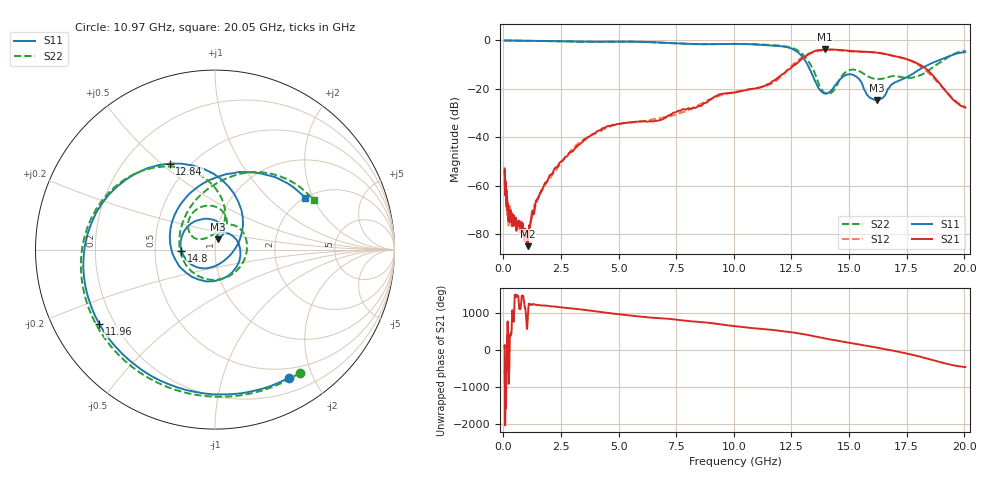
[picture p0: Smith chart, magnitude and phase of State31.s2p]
# Hz S DB R 50
!freq MagS11 AngS11 MagS21 AngS21 MagS12 AngS12 MagS22 AngS22
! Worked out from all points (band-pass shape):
!   1601 points, 50 MHz to 20.05 GHz, reference 50 ohm
!   highest |S21| = -3.69 dB at 13.94 GHz (marker M1); lowest = -85.1 dB at 1.047 GHz (marker M2)
!   |S21| within 3 dB of the highest: 13.1 GHz to 17.09 GHz (3.995 GHz wide, 26.5 % of centre)
!   lowest |S11| = -24.6 dB at 16.19 GHz (marker M3), VSWR 1.12, Z = 51.1 + j5.85 ohm
!   |S11| at or under -10 dB: 13.2 GHz to 18.45 GHz (5.254 GHz wide, 33.2 % of centre)
!   |S22| runs from -22.1 to 0.0 dB; largest |S21 - S12| = 0.044
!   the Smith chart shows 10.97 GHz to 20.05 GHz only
!   S11 on the Smith chart (normalised r, x): 10.97 GHz: 0.37, -1.66; 11.96 GHz: 0.14, -0.29; 12.84 GHz: 0.39, +0.53; 14.8 GHz: 0.69, -0.01; 20.05 GHz: 2.00, +1.74
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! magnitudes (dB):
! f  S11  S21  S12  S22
! 50 MHz  0.0  -55.4  -52.4  0.0
! 58.96 MHz  0.0  -55.1  -58.3  0.0
! 78.67 MHz  0.0  -62.8  -59.4  0.0
! 87.38 MHz  0.0  -59.9  -58.9  0.0
! 135.9 MHz  0.0  -66.6  -66.5  0.0
! 222.1 MHz  0.0  -74.2  -76.0  0.0
! 253.2 MHz  0.0  -71.2  -69.1  0.0
! 369.6 MHz  0.0  -76.4  -73.3  0.0
! 457.6 MHz  0.0  -73.5  -75.3  0.0
! 1.005 GHz  -0.1  -82.7  -80.7  -0.1
! 1.047 GHz  -0.1  -85.1  -81.0  -0.1
! 2.722 GHz  -0.3  -48.1  -48.0  -0.4
! 4.397 GHz  -0.5  -36.1  -36.5  -0.6
! 7.402 GHz  -1.1  -29.8  -30.8  -1.1
! 10.97 GHz  -1.7  -19.8  -19.7  -1.6
! 11.96 GHz  -2.3  -15.1  -15.7  -2.1
! 12.84 GHz  -5.3  -8.6  -7.8  -4.5
! 13.94 GHz  -22.0  -3.7  -3.9  -21.6
! 14.8 GHz  -14.6  -4.1  -4.3  -13.5
! 16.19 GHz  -24.6  -5.0  -5.0  -16.0
! 18.05 GHz  -12.0  -9.9  -10.4  -14.5
! 20.05 GHz  -4.7  -27.8  -27.5  -4.2
